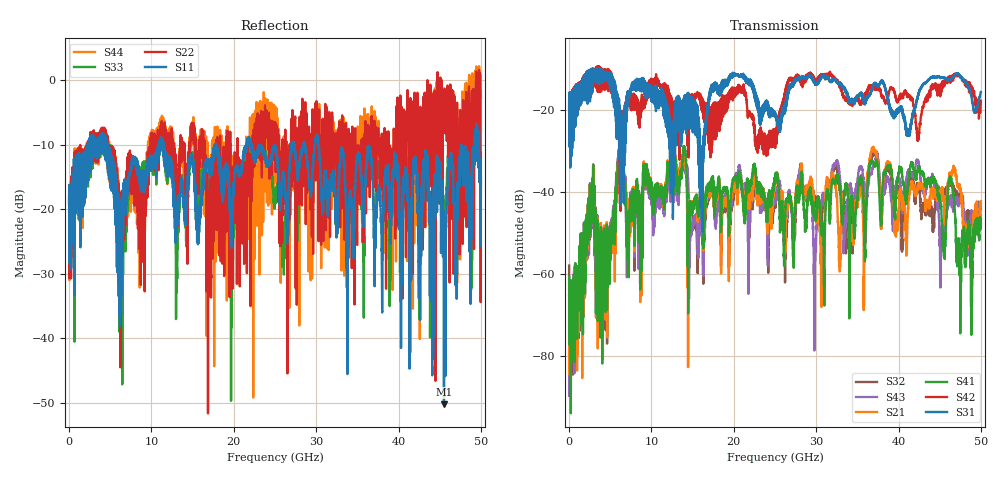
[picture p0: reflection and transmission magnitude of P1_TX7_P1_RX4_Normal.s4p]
!Keysight Technologies,N5225B,MY57041031,A.13.20.10
!Date: Friday, May 31, 2019 11:19:28
!Correction: S11(Full 4 Port(1,2,3,4))
!S12(Full 4 Port(1,2,3,4))
!S13(Full 4 Port(1,2,3,4))
!S14(Full 4 Port(1,2,3,4))
!S21(Full 4 Port(1,2,3,4))
!S22(Full 4 Port(1,2,3,4))
!S23(Full 4 Port(1,2,3,4))
!S24(Full 4 Port(1,2,3,4))
!S31(Full 4 Port(1,2,3,4))
!S32(Full 4 Port(1,2,3,4))
!S33(Full 4 Port(1,2,3,4))
!S34(Full 4 Port(1,2,3,4))
!S41(Full 4 Port(1,2,3,4))
!S42(Full 4 Port(1,2,3,4))
!S43(Full 4 Port(1,2,3,4))
!S44(Full 4 Port(1,2,3,4))
!S4P File: Measurements: <S11,S12,S13,S14>,
!<S21,S22,S23,S24>,
!<S31,S32,S33,S34>,
!<S41,S42,S43,S44>:
# Hz S  dB  R 50.0
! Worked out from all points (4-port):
!   5000 points, 10 MHz to 50 GHz, reference 50 ohm
!   strongest paths, dB at 10 MHz, 12.51 GHz, 25.01 GHz, 37.51 GHz, 50 GHz:
!     S31: -19.4, -39.5, -20.8, -14.0, -15.5
!     S42: -19.4, -19.3, -26.3, -15.0, -17.6
!     S41: -60.7, -38.0, -37.8, -34.1, -47.7
!     S21: -65.0, -37.0, -38.6, -33.7, -42.2
!     S43: -62.8, -39.1, -42.7, -31.7, -44.1
!     S32: -57.9, -37.8, -43.7, -31.9, -46.4
!   lowest |S11| = -50.2 dB at 45.52 GHz (marker M1), VSWR 1.01, Z = 49.8 + j0.206 ohm
!   |S11| at or under -10 dB: 4.613 GHz to 10.86 GHz (6.246 GHz wide, 80.7 % of centre); 11.46 GHz to 17.73 GHz (6.279 GHz wide, 43 % of centre); 30.28 GHz to 47.61 GHz (17.33 GHz wide, 44.5 % of centre)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
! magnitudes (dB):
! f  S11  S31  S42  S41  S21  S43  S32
! 10 MHz  -19.2  -19.4  -19.4  -60.7  -65.0  -62.8  -57.9
! 6.26 GHz  -21.5  -21.0  -28.9  -29.4  -29.9  -28.9  -29.3
! 15.55 GHz  -25.1  -20.7  -16.0  -42.8  -45.4  -49.7  -54.5
! 30.7 GHz  -17.5  -11.5  -11.2  -49.4  -55.1  -42.2  -45.6
! 37.31 GHz  -20.6  -13.5  -14.6  -32.5  -30.4  -31.2  -30.3
! 45.52 GHz  -50.2  -12.0  -13.3  -55.7  -43.0  -52.7  -41.9
! 50 GHz  -15.5  -15.5  -17.6  -47.7  -42.2  -44.1  -46.4
